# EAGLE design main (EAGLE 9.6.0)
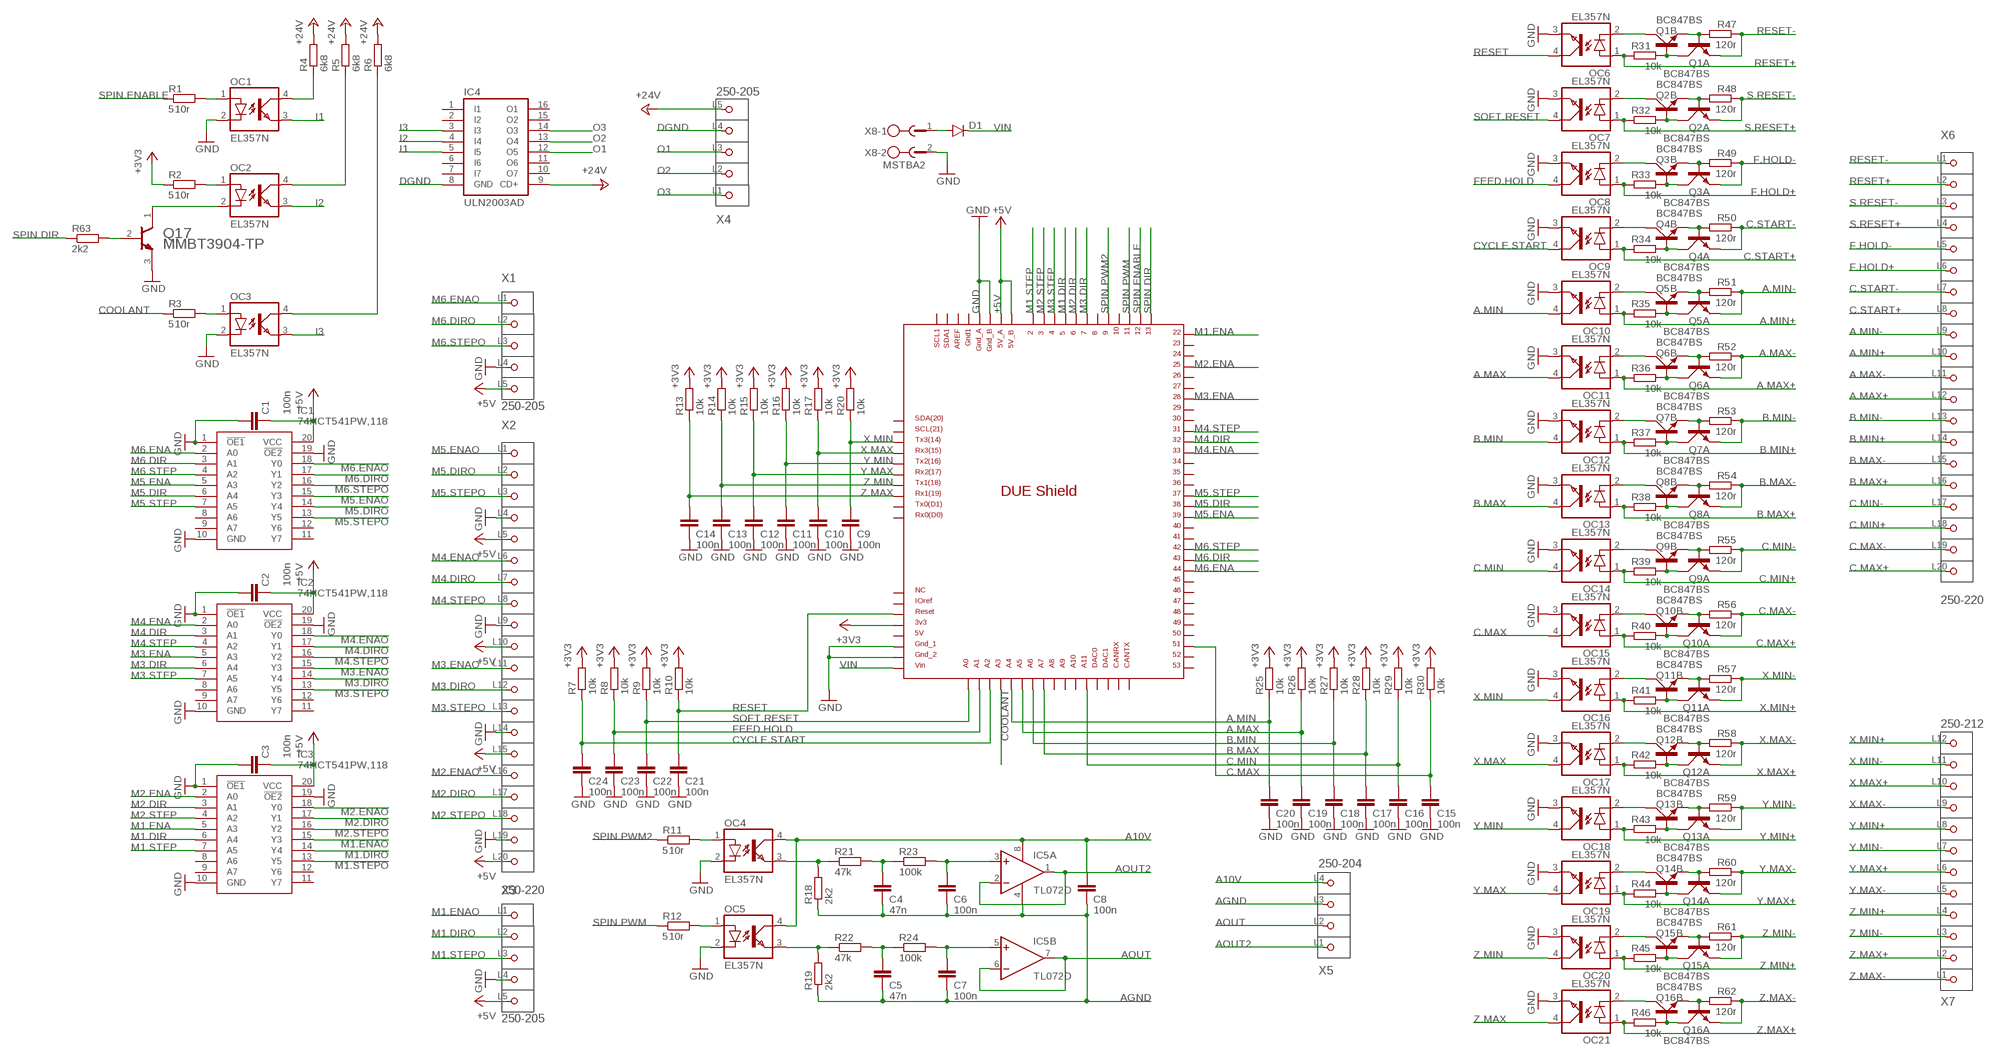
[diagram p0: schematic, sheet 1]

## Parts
C1  100n  CAP_0402  [0402]
C2  100n  CAP_0402  [0402]
C3  100n  CAP_0402  [0402]
C4  47n  CAP_0402  [0402]
C5  47n  CAP_0402  [0402]
C6  100n  CAP_0402  [0402]
C7  100n  CAP_0402  [0402]
C8  100n  CAP_0402  [0402]
C9  100n  CAP_0402  [0402]
C10  100n  CAP_0402  [0402]
C11  100n  CAP_0402  [0402]
C12  100n  CAP_0402  [0402]
C13  100n  CAP_0402  [0402]
C14  100n  CAP_0402  [0402]
C15  100n  CAP_0402  [0402]
C16  100n  CAP_0402  [0402]
C17  100n  CAP_0402  [0402]
C18  100n  CAP_0402  [0402]
C19  100n  CAP_0402  [0402]
C20  100n  CAP_0402  [0402]
C21  100n  CAP_0402  [0402]
C22  100n  CAP_0402  [0402]
C23  100n  CAP_0402  [0402]
C24  100n  CAP_0402  [0402]
D1  DIODE-DO214AC  [DO214AC]
IC1  74HCT541PW,118  [SOP65P640X110-20N]
IC2  74HCT541PW,118  [SOP65P640X110-20N]
IC3  74HCT541PW,118  [SOP65P640X110-20N]
IC4  ULN2003AD  [SO16]
IC5  TL072D  [SO08]
MCU1  DUE(NORMAL)  [DUE(NORMAL)]
OC1  EL357N  [SOP4]
OC2  EL357N  [SOP4]
OC3  EL357N  [SOP4]
OC4  EL357N  [SOP4]
OC5  EL357N  [SOP4]
OC6  EL357N  [SOP4]
OC7  EL357N  [SOP4]
OC8  EL357N  [SOP4]
OC9  EL357N  [SOP4]
OC10  EL357N  [SOP4]
OC11  EL357N  [SOP4]
OC12  EL357N  [SOP4]
OC13  EL357N  [SOP4]
OC14  EL357N  [SOP4]
OC15  EL357N  [SOP4]
OC16  EL357N  [SOP4]
OC17  EL357N  [SOP4]
OC18  EL357N  [SOP4]
OC19  EL357N  [SOP4]
OC20  EL357N  [SOP4]
OC21  EL357N  [SOP4]
Q1  BC847BS  [SOT363_PHILIPS]
Q2  BC847BS  [SOT363_PHILIPS]
Q3  BC847BS  [SOT363_PHILIPS]
Q4  BC847BS  [SOT363_PHILIPS]
Q5  BC847BS  [SOT363_PHILIPS]
Q6  BC847BS  [SOT363_PHILIPS]
Q7  BC847BS  [SOT363_PHILIPS]
Q8  BC847BS  [SOT363_PHILIPS]
Q9  BC847BS  [SOT363_PHILIPS]
Q10  BC847BS  [SOT363_PHILIPS]
Q11  BC847BS  [SOT363_PHILIPS]
Q12  BC847BS  [SOT363_PHILIPS]
Q13  BC847BS  [SOT363_PHILIPS]
Q14  BC847BS  [SOT363_PHILIPS]
Q15  BC847BS  [SOT363_PHILIPS]
Q16  BC847BS  [SOT363_PHILIPS]
Q17  MICRO_COMMERCIAL_MMBT3904-TPMICRO_COMMERCIAL_MMBT3904-TP_0_0  [MICRO_COMMERCIAL_MMBT3904-TP_0]
R1  510r  R-EU_R0402  [R0402]
R2  510r  R-EU_R0402  [R0402]
R3  510r  R-EU_R0402  [R0402]
R4  6k8  R-EU_R0603  [R0603]
R5  6k8  R-EU_R0603  [R0603]
R6  6k8  R-EU_R0603  [R0603]
R7  10k  R-EU_R0402  [R0402]
R8  10k  R-EU_R0402  [R0402]
R9  10k  R-EU_R0402  [R0402]
R10  10k  R-EU_R0402  [R0402]
R11  510r  R-EU_R0402  [R0402]
R12  510r  R-EU_R0402  [R0402]
R13  10k  R-EU_R0402  [R0402]
R14  10k  R-EU_R0402  [R0402]
R15  10k  R-EU_R0402  [R0402]
R16  10k  R-EU_R0402  [R0402]
R17  10k  R-EU_R0402  [R0402]
R18  2k2  R-EU_R0402  [R0402]
R19  2k2  R-EU_R0402  [R0402]
R20  10k  R-EU_R0402  [R0402]
R21  47k  R-EU_R0402  [R0402]
R22  47k  R-EU_R0402  [R0402]
R23  100k  R-EU_R0402  [R0402]
R24  100k  R-EU_R0402  [R0402]
R25  10k  R-EU_R0402  [R0402]
R26  10k  R-EU_R0402  [R0402]
R27  10k  R-EU_R0402  [R0402]
R28  10k  R-EU_R0402  [R0402]
R29  10k  R-EU_R0402  [R0402]
R30  10k  R-EU_R0402  [R0402]
R31  10k  R-EU_R0402  [R0402]
R32  10k  R-EU_R0402  [R0402]
R33  10k  R-EU_R0402  [R0402]
R34  10k  R-EU_R0402  [R0402]
R35  10k  R-EU_R0402  [R0402]
R36  10k  R-EU_R0402  [R0402]
R37  10k  R-EU_R0402  [R0402]
R38  10k  R-EU_R0402  [R0402]
R39  10k  R-EU_R0402  [R0402]
R40  10k  R-EU_R0402  [R0402]
R41  10k  R-EU_R0402  [R0402]
R42  10k  R-EU_R0402  [R0402]
R43  10k  R-EU_R0402  [R0402]
R44  10k  R-EU_R0402  [R0402]
R45  10k  R-EU_R0402  [R0402]
R46  10k  R-EU_R0402  [R0402]
R47  120r  R-EU_R0402  [R0402]
R48  120r  R-EU_R0402  [R0402]
R49  120r  R-EU_R0402  [R0402]
R50  120r  R-EU_R0402  [R0402]
R51  120r  R-EU_R0402  [R0402]
R52  120r  R-EU_R0402  [R0402]
R53  120r  R-EU_R0402  [R0402]
R54  120r  R-EU_R0402  [R0402]
R55  120r  R-EU_R0402  [R0402]
R56  120r  R-EU_R0402  [R0402]
R57  120r  R-EU_R0402  [R0402]
R58  120r  R-EU_R0402  [R0402]
R59  120r  R-EU_R0402  [R0402]
R60  120r  R-EU_R0402  [R0402]
R61  120r  R-EU_R0402  [R0402]
R62  120r  R-EU_R0402  [R0402]
R63  2k2  R-EU_R0402  [R0402]
X1  250-205  [P-250-205]
X2  250-220  [P-250-220]
X3  250-205  [P-250-205]
X4  250-205  [P-250-205]
X5  250-204  [P-250-204]
X6  250-220  [P-250-220]
X7  250-212  [P-250-212]
X8  MSTBA2  [MSTBA2]

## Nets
+3V3 [power1]: MCU1.3V3 R2.1 R7.2 R8.2 R9.2 R10.2 R13.2 R14.2 R15.2 R16.2 R17.2 R20.2 R25.2 R26.2 R27.2 R28.2 R29.2 R30.2
+5V [power1]: C1.2 C2.2 C3.2 IC1.20(VCC) IC2.20(VCC) IC3.20(VCC) MCU1.5V_A MCU1.5V_B X1.L5(P5) X2.L5(P5) X2.L10(P10) X2.L15(P15) X2.L20(P20) X3.L5(P5)
+24V [power1]: IC4.9(CD+) R4.2 R5.2 R6.2 X4.L5(P5)
A10V [signal1]: C8.1 IC5.8(P:V+) OC4.4(COL) OC5.4(COL) X5.L4(P4)
A.MAX [signal1]: C19.1 MCU1.A5 OC11.4(COL) R26.1
A.MAX+ [signal1]: OC11.1(A) R36.2 X6.L12(P12)
A.MAX- [signal1]: Q6.1(A:E) R52.1 X6.L11(P11)
A.MIN [signal1]: C20.1 MCU1.A4 OC10.4(COL) R25.1
A.MIN+ [signal1]: OC10.1(A) R35.2 X6.L10(P10)
A.MIN- [signal1]: Q5.1(A:E) R51.1 X6.L9(P9)
AGND [signal1]: C4.2 C5.2 C6.2 C7.2 C8.2 IC5.4(P:V-) R18.1 R19.1 X5.L3(P3)
AOUT [signal1]: IC5.6(B:-IN) IC5.7(B:OUT) X5.L2(P2)
AOUT2 [signal1]: IC5.1(A:OUT) IC5.2(A:-IN) X5.L1(P1)
B.MAX [signal1]: C17.1 MCU1.A7 OC13.4(COL) R28.1
B.MAX+ [signal1]: OC13.1(A) R38.2 X6.L16(P16)
B.MAX- [signal1]: Q8.1(A:E) R54.1 X6.L15(P15)
B.MIN [signal1]: C18.1 MCU1.A6 OC12.4(COL) R27.1
B.MIN+ [signal1]: OC12.1(A) R37.2 X6.L14(P14)
B.MIN- [signal1]: Q7.1(A:E) R53.1 X6.L13(P13)
C.MAX [signal1]: C15.1 MCU1.51 OC15.4(COL) R30.1
C.MAX+ [signal1]: OC15.1(A) R40.2 X6.L20(P20)
C.MAX- [signal1]: Q10.1(A:E) R56.1 X6.L19(P19)
C.MIN [signal1]: C16.1 MCU1.A11 OC14.4(COL) R29.1
C.MIN+ [signal1]: OC14.1(A) R39.2 X6.L18(P18)
C.MIN- [signal1]: Q9.1(A:E) R55.1 X6.L17(P17)
C.START+ [signal1]: OC9.1(A) R34.2 X6.L8(P8)
C.START- [signal1]: Q4.1(A:E) R50.1 X6.L7(P7)
COOLANT [signal1]: MCU1.A3 R3.1
CYCLE.START [signal1]: C24.1 MCU1.A2 OC9.4(COL) R7.1
DGND [power1]: IC4.8(GND) X4.L4(P4)
F.HOLD+ [signal1]: OC8.1(A) R33.2 X6.L6(P6)
F.HOLD- [signal1]: Q3.1(A:E) R49.1 X6.L5(P5)
FEED.HOLD [signal1]: C23.1 MCU1.A1 OC8.4(COL) R8.1
GND: C1.1 C2.1 C3.1 C9.2 C10.2 C11.2 C12.2 C13.2 C14.2 C15.2 C16.2 C17.2 C18.2 C19.2 C20.2 C21.2 C22.2 C23.2 C24.2 IC1.1(!OE1) IC1.10(GND) IC1.19(!OE2) IC2.1(!OE1) IC2.10(GND) IC2.19(!OE2) IC3.1(!OE1) IC3.10(GND) IC3.19(!OE2) MCU1.GND_1 MCU1.GND_2 MCU1.GND_A MCU1.GND_B OC1.2(C) OC3.2(C) OC4.2(C) OC5.2(C) OC6.3(EMIT) OC7.3(EMIT) OC8.3(EMIT) OC9.3(EMIT) OC10.3(EMIT) OC11.3(EMIT) OC12.3(EMIT) OC13.3(EMIT) OC14.3(EMIT) OC15.3(EMIT) OC16.3(EMIT) OC17.3(EMIT) OC18.3(EMIT) OC19.3(EMIT) OC20.3(EMIT) OC21.3(EMIT) Q17.3(E) X1.L4(P4) X2.L4(P4) X2.L9(P9) X2.L14(P14) X2.L19(P19) X3.L4(P4) X8.2
I1 [signal1]: IC4.5(I5) OC1.3(EMIT)
I2 [signal1]: IC4.4(I4) OC2.3(EMIT)
I3 [signal1]: IC4.3(I3) OC3.3(EMIT)
M1.DIR [signal1]: IC3.6(A4) MCU1.5
M1.DIRO [signal1]: IC3.14(Y4) X3.L2(P2)
M1.ENA [signal1]: IC3.5(A3) MCU1.22
M1.ENAO [signal1]: IC3.15(Y3) X3.L1(P1)
M1.STEP [signal1]: IC3.7(A5) MCU1.2
M1.STEPO [signal1]: IC3.13(Y5) X3.L3(P3)
M2.DIR [signal1]: IC3.3(A1) MCU1.6
M2.DIRO [signal1]: IC3.17(Y1) X2.L17(P17)
M2.ENA [signal1]: IC3.2(A0) MCU1.25
M2.ENAO [signal1]: IC3.18(Y0) X2.L16(P16)
M2.STEP [signal1]: IC3.4(A2) MCU1.3
M2.STEPO [signal1]: IC3.16(Y2) X2.L18(P18)
M3.DIR [signal1]: IC2.6(A4) MCU1.7
M3.DIRO [signal1]: IC2.14(Y4) X2.L12(P12)
M3.ENA [signal1]: IC2.5(A3) MCU1.28
M3.ENAO [signal1]: IC2.15(Y3) X2.L11(P11)
M3.STEP [signal1]: IC2.7(A5) MCU1.4
M3.STEPO [signal1]: IC2.13(Y5) X2.L13(P13)
M4.DIR [signal1]: IC2.3(A1) MCU1.32
M4.DIRO [signal1]: IC2.17(Y1) X2.L7(P7)
M4.ENA [signal1]: IC2.2(A0) MCU1.33
M4.ENAO [signal1]: IC2.18(Y0) X2.L6(P6)
M4.STEP [signal1]: IC2.4(A2) MCU1.31
M4.STEPO [signal1]: IC2.16(Y2) X2.L8(P8)
M5.DIR [signal1]: IC1.6(A4) MCU1.38
M5.DIRO [signal1]: IC1.14(Y4) X2.L2(P2)
M5.ENA [signal1]: IC1.5(A3) MCU1.39
M5.ENAO [signal1]: IC1.15(Y3) X2.L1(P1)
M5.STEP [signal1]: IC1.7(A5) MCU1.37
M5.STEPO [signal1]: IC1.13(Y5) X2.L3(P3)
M6.DIR [signal1]: IC1.3(A1) MCU1.43
M6.DIRO [signal1]: IC1.17(Y1) X1.L2(P2)
M6.ENA [signal1]: IC1.2(A0) MCU1.44
M6.ENAO [signal1]: IC1.18(Y0) X1.L1(P1)
M6.STEP [signal1]: IC1.4(A2) MCU1.42
M6.STEPO [signal1]: IC1.16(Y2) X1.L3(P3)
N$2 [signal1]: Q16.5(B:B) Q16.6(A:C) R46.1
N$3 [signal1]: Q16.2(A:B) Q16.4(B:E) R62.2
N$4 [signal1]: OC21.2(C) Q16.3(B:C)
N$5 [signal1]: Q15.5(B:B) Q15.6(A:C) R45.1
N$6 [signal1]: Q15.2(A:B) Q15.4(B:E) R61.2
N$7 [signal1]: OC20.2(C) Q15.3(B:C)
N$8 [signal1]: Q14.5(B:B) Q14.6(A:C) R44.1
N$9 [signal1]: Q14.2(A:B) Q14.4(B:E) R60.2
N$10 [signal1]: OC19.2(C) Q14.3(B:C)
N$11 [signal1]: Q13.5(B:B) Q13.6(A:C) R43.1
N$12 [signal1]: Q13.2(A:B) Q13.4(B:E) R59.2
N$13 [signal1]: OC18.2(C) Q13.3(B:C)
N$14 [signal1]: Q12.5(B:B) Q12.6(A:C) R42.1
N$15 [signal1]: Q12.2(A:B) Q12.4(B:E) R58.2
N$16 [signal1]: OC17.2(C) Q12.3(B:C)
N$17 [signal1]: Q11.5(B:B) Q11.6(A:C) R41.1
N$18 [signal1]: Q11.2(A:B) Q11.4(B:E) R57.2
N$19 [signal1]: OC15.2(C) Q10.3(B:C)
N$20 [signal1]: Q10.5(B:B) Q10.6(A:C) R40.1
N$21 [signal1]: Q10.2(A:B) Q10.4(B:E) R56.2
N$22 [signal1]: OC16.2(C) Q11.3(B:C)
N$23 [signal1]: Q4.5(B:B) Q4.6(A:C) R34.1
N$24 [signal1]: Q9.5(B:B) Q9.6(A:C) R39.1
N$25 [signal1]: Q9.2(A:B) Q9.4(B:E) R55.2
N$26 [signal1]: OC4.3(EMIT) R18.2 R21.1
N$27 [signal1]: C5.1 R22.2 R24.1
N$28 [signal1]: OC14.2(C) Q9.3(B:C)
N$29 [signal1]: Q8.5(B:B) Q8.6(A:C) R38.1
N$30 [signal1]: Q8.2(A:B) Q8.4(B:E) R54.2
N$31 [signal1]: C4.1 R21.2 R23.1
N$32 [signal1]: C6.1 IC5.3(A:+IN) R23.2
N$33 [signal1]: OC13.2(C) Q8.3(B:C)
N$34 [signal1]: Q7.5(B:B) Q7.6(A:C) R37.1
N$35 [signal1]: Q7.2(A:B) Q7.4(B:E) R53.2
N$36 [signal1]: C7.1 IC5.5(B:+IN) R24.2
N$37 [signal1]: OC4.1(A) R11.2
N$38 [signal1]: OC12.2(C) Q7.3(B:C)
N$39 [signal1]: Q6.5(B:B) Q6.6(A:C) R36.1
N$40 [signal1]: Q6.2(A:B) Q6.4(B:E) R52.2
N$41 [signal1]: OC5.3(EMIT) R19.2 R22.1
N$42 [signal1]: OC5.1(A) R12.2
N$43 [signal1]: OC11.2(C) Q6.3(B:C)
N$44 [signal1]: Q5.5(B:B) Q5.6(A:C) R35.1
N$45 [signal1]: Q5.2(A:B) Q5.4(B:E) R51.2
N$46 [signal1]: Q4.2(A:B) Q4.4(B:E) R50.2
N$47 [signal1]: OC9.2(C) Q4.3(B:C)
N$48 [signal1]: OC10.2(C) Q5.3(B:C)
N$49 [signal1]: Q3.5(B:B) Q3.6(A:C) R33.1
N$50 [signal1]: Q3.2(A:B) Q3.4(B:E) R49.2
N$51 [signal1]: OC8.2(C) Q3.3(B:C)
N$52 [signal1]: Q2.5(B:B) Q2.6(A:C) R32.1
N$53 [signal1]: Q2.2(A:B) Q2.4(B:E) R48.2
N$54 [signal1]: OC7.2(C) Q2.3(B:C)
N$55 [signal1]: Q1.5(B:B) Q1.6(A:C) R31.1
N$56 [signal1]: Q1.2(A:B) Q1.4(B:E) R47.2
N$57 [signal1]: OC6.2(C) Q1.3(B:C)
N$58 [signal1]: OC1.1(A) R1.2
N$59 [signal1]: OC2.1(A) R2.2
N$60 [signal1]: OC3.1(A) R3.2
N$61 [signal1]: OC1.4(COL) R4.1
N$62 [signal1]: OC2.4(COL) R5.1
N$63 [signal1]: OC3.4(COL) R6.1
N$64: OC2.2(C) Q17.1(C)
N$65: Q17.2(B) R63.2
N$66 [power1]: D1.A X8.1
O1 [power1]: IC4.12(O5) X4.L3(P3)
O2 [power1]: IC4.13(O4) X4.L2(P2)
O3 [power1]: IC4.14(O3) X4.L1(P1)
RESET [signal1]: C21.1 MCU1.RESET OC6.4(COL) R10.1
RESET+ [signal1]: OC6.1(A) R31.2 X6.L2(P2)
RESET- [signal1]: Q1.1(A:E) R47.1 X6.L1(P1)
S.RESET+ [signal1]: OC7.1(A) R32.2 X6.L4(P4)
S.RESET- [signal1]: Q2.1(A:E) R48.1 X6.L3(P3)
SOFT.RESET [signal1]: C22.1 MCU1.A0 OC7.4(COL) R9.1
SPIN.DIR [signal1]: MCU1.13 R63.1
SPIN.ENABLE [signal1]: MCU1.12 R1.1
SPIN.PWM [signal1]: MCU1.11 R12.1
SPIN.PWM2 [signal1]: MCU1.9 R11.1
VIN [power1]: D1.C MCU1.VIN
X.MAX [signal1]: C10.1 MCU1.RX3 OC17.4(COL) R17.1
X.MAX+ [signal1]: OC17.1(A) R42.2 X7.L10(P10)
X.MAX- [signal1]: Q12.1(A:E) R58.1 X7.L9(P9)
X.MIN [signal1]: C9.1 MCU1.TX3 OC16.4(COL) R20.1
X.MIN+ [signal1]: OC16.1(A) R41.2 X7.L12(P12)
X.MIN- [signal1]: Q11.1(A:E) R57.1 X7.L11(P11)
Y.MAX [signal1]: C12.1 MCU1.RX2 OC19.4(COL) R15.1
Y.MAX+ [signal1]: OC19.1(A) R44.2 X7.L6(P6)
Y.MAX- [signal1]: Q14.1(A:E) R60.1 X7.L5(P5)
Y.MIN [signal1]: C11.1 MCU1.TX2 OC18.4(COL) R16.1
Y.MIN+ [signal1]: OC18.1(A) R43.2 X7.L8(P8)
Y.MIN- [signal1]: Q13.1(A:E) R59.1 X7.L7(P7)
Z.MAX [signal1]: C14.1 MCU1.RX1 OC21.4(COL) R13.1
Z.MAX+ [signal1]: OC21.1(A) R46.2 X7.L2(P2)
Z.MAX- [signal1]: Q16.1(A:E) R62.1 X7.L1(P1)
Z.MIN [signal1]: C13.1 MCU1.TX1 OC20.4(COL) R14.1
Z.MIN+ [signal1]: OC20.1(A) R45.2 X7.L4(P4)
Z.MIN- [signal1]: Q15.1(A:E) R61.1 X7.L3(P3)
Unconnected: IC1.8(A6) IC1.9(A7) IC1.11(Y7) IC1.12(Y6) IC2.8(A6) IC2.9(A7) IC2.11(Y7) IC2.12(Y6) IC3.8(A6) IC3.9(A7) IC3.11(Y7) IC3.12(Y6) IC4.1(I1) IC4.2(I2) IC4.6(I6) IC4.7(I7) IC4.10(O7) IC4.11(O6) IC4.15(O2) IC4.16(O1) MCU1.5V MCU1.8 MCU1.10 MCU1.23 MCU1.24 MCU1.26 MCU1.27 MCU1.29 MCU1.30 MCU1.34 MCU1.35 MCU1.36 MCU1.40 MCU1.41 MCU1.45 MCU1.46 MCU1.47 MCU1.48 MCU1.49 MCU1.50 MCU1.52 MCU1.53 MCU1.A8 MCU1.A9 MCU1.A10 MCU1.AREF MCU1.CANRX MCU1.CANTX MCU1.DAC0 MCU1.DAC1 MCU1.GND1 MCU1.IOREF MCU1.NC MCU1.RX0 MCU1.SCL MCU1.SCL1 MCU1.SDA MCU1.SDA1 MCU1.TX0

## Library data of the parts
C1-C24 = Perfect_0402:CAP_0402: 0402 (1005 Metric)
D1 = mydiode:DIODE-: DIODE
IC1-IC3 = SamacSys_Parts:74HCT541PW,118: 74HC(T)541 - Octal buffer/line driver; 3-state@en-us Source: Datasheet; DESCRIPTION: 74HC(T)541 - Octal buffer/line driver; 3-state@en-us; HEIGHT: 1.1mm; MANUFACTURER_NAME: Nexperia; MANUFACTURER_PART_NUMBER: 74HCT541PW,118; MOUSER_PART_NUMBER: 771-74HCT541PW-T; MOUSER_PRICE-STOCK: https://www.mouser.com/Search/Refine.aspx?Keyword=771-74HCT541PW-T
IC4 = uln-udn:ULN2003A: DRIVER ARRAY
IC5 = linear:TL072: OP AMP
MCU1 = DUElib130425:DUE(NORMAL)
OC1-OC21 = el357n:EL357N
Q1-Q16 = transistor-small-signal:BC847BS: NPN general purpose double transistor Source: http://www.farnell.com/datasheets/2466.pdf
Q17 = Micro Commercial - MMBT3904-TP:MICRO_COMMERCIAL_MMBT3904-TP: TRANS NPN 40V 0.2A SOT23; CENTROID_NOT_SPECIFIED: No; COLLECTOR_EMITTER_BREAKDOWN_VOLTAGE: 40V; COLLECTOR_EMITTER_SATURATION_VOLTAGE: 0.2V; DATASHEET: http://www.mccsemi.com/up_pdf/MMBT3904(SOT-23)-F.pdf; DEVICE_CLASS_L1: Discrete Semiconductors; DEVICE_CLASS_L2: Transistors; DEVICE_CLASS_L3: BJTs; DIGIKEY_DESCRIPTION: TRANS NPN 40V 0.2A SOT23; DIGIKEY_PART_NUMBER: MMBT3904TPMSCT-ND; GAIN_BANDWIDTH_PRODUCT: 300MHz; HEIGHT: 1.12mm; HFE_MIN: 100; LEAD_FREE: yes; MAX_COLLECTOR_CURRENT: 200mA; MAX_JUNCTION_TEMP: +150°C; MF: Micro Commercial; MFG_PACKAGE_IDENT: SOT-23; MFG_PACKAGE_IDENT_DATE: 0; MFG_PACKAGE_IDENT_REV: 0; MOUSER_DESCRIPTION: Bipolar Transistors - BJT 40V; MOUSER_PART_NUMBER: 833-MMBT3904-TP; MPN: MMBT3904-TP; NUMBER_OF_ELEMENTS: 1; NUMBER_OF_NPN: 1; NUMBER_OF_PNP: 0; PACKAGE: SOT23-3; POWER_DISSIPATION: 350mW; PREFIX: Q; ROHS: yes; STANDOFF_HEIGHT: 0.013mm; TEMPERATURE_RANGE_HIGH: +150°C; TEMPERATURE_RANGE_LOW: -55°C; VERIFICATION_VERSION: 0.0.0.1
R1-R63 = rcl:R-EU_: RESISTOR, European symbol; SPICEPREFIX: R
X1 X3 X4 = con-wago_250:250-205: Serie 250, 1-Leiter-Klemmenleiste für Leiterplatten 1 Lötstift/Pol versetzt / Series 250, 1-conductor PCB terminal strip 1 solder pin/pole, staggered Polzahl / Pole No.: 5 Rastermaß / Pitch: 3.5 - 3.5 mm Bemessungsspannung / Rated Voltage: 320 V Nennstrom / Nominal Current: 8 A Leiterquerschnitt /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
X2 X6 = con-wago_250:250-220: Serie 250, 1-Leiter-Klemmenleiste für Leiterplatten 1 Lötstift/Pol versetzt / Series 250, 1-conductor PCB terminal strip 1 solder pin/pole, staggered Polzahl / Pole No.: 20 Rastermaß / Pitch: 3.5 - 3.5 mm Bemessungsspannung / Rated Voltage: 320 V Nennstrom / Nominal Current: 8 A Leiterquerschnitt /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
X5 = con-wago_250:250-204: Serie 250, 1-Leiter-Klemmenleiste für Leiterplatten 1 Lötstift/Pol versetzt / Series 250, 1-conductor PCB terminal strip 1 solder pin/pole, staggered Polzahl / Pole No.: 4 Rastermaß / Pitch: 3.5 - 3.5 mm Bemessungsspannung / Rated Voltage: 320 V Nennstrom / Nominal Current: 8 A Leiterquerschnitt /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
X7 = con-wago_250:250-212: Serie 250, 1-Leiter-Klemmenleiste für Leiterplatten 1 Lötstift/Pol versetzt / Series 250, 1-conductor PCB terminal strip 1 solder pin/pole, staggered Polzahl / Pole No.: 12 Rastermaß / Pitch: 3.5 - 3.5 mm Bemessungsspannung / Rated Voltage: 320 V Nennstrom / Nominal Current: 8 A Leiterquerschnitt /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
X8 = con-phoenix-508:MSTBA2: PHOENIX; MF: FARNELL; MPN: 1757242; OC_FARNELL: 3705171; OC_NEWARK: 71C4161

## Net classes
0 default: clearance 0.254 mm
1 power1: width 0.457 mm
2 signal1: width 0.305 mm

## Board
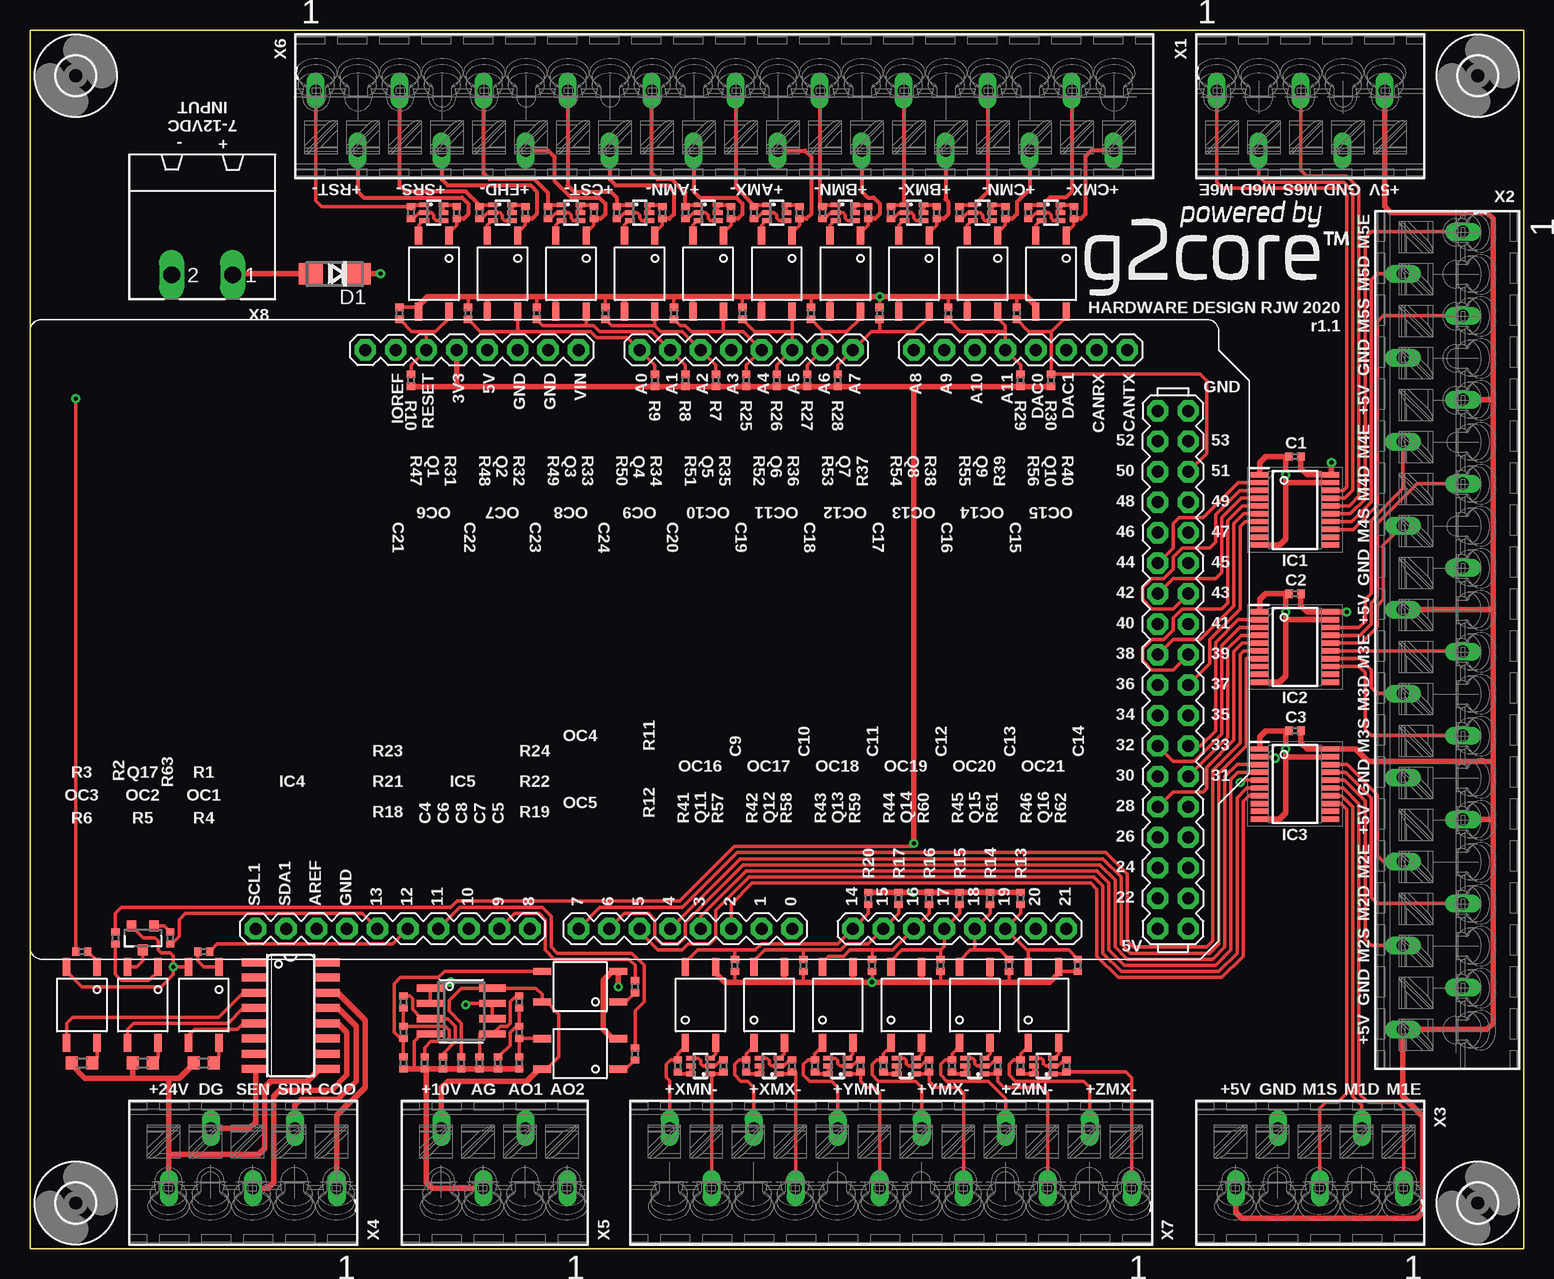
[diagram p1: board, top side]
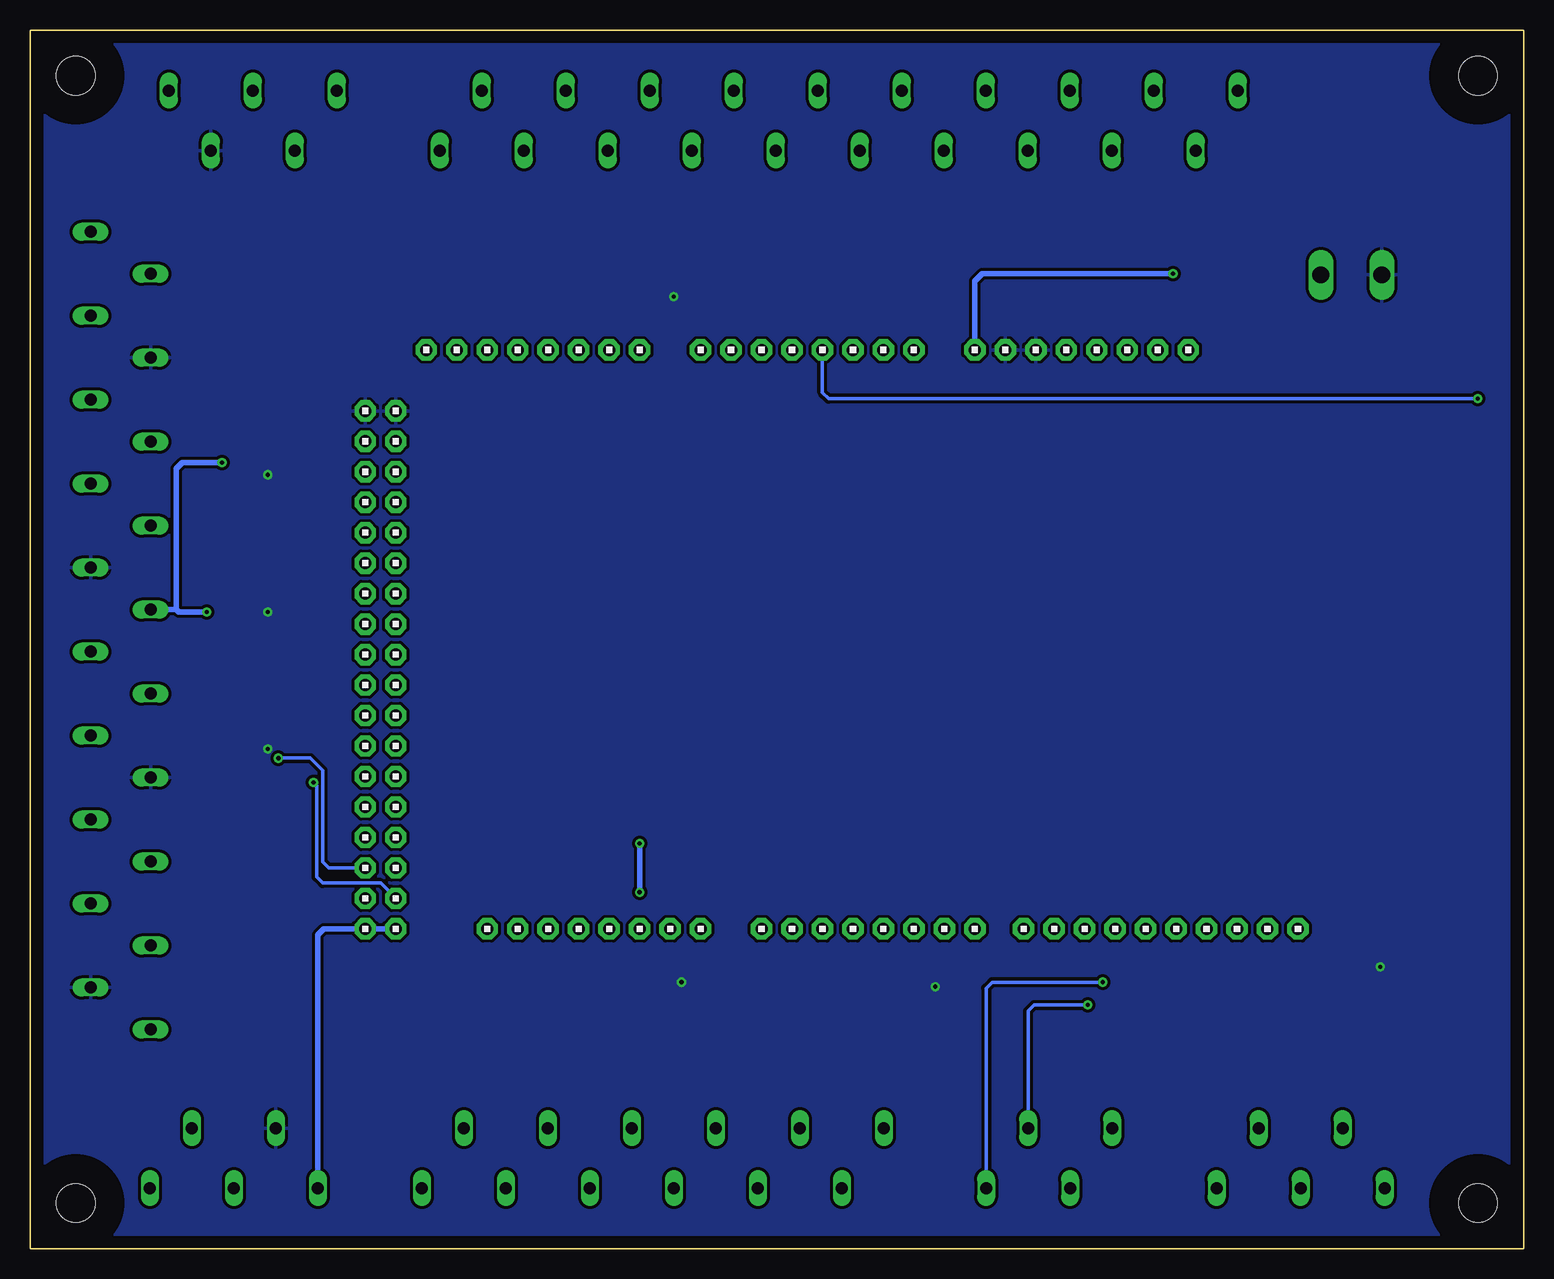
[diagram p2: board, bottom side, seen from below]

Size 124.46 x 101.6 mm. Coordinates in mm from the lower left corner, seen from the top.
Outline: 0,101.6 124.46,101.6 124.46,0 0,0 0,101.6
Copper layers (1*16): Top 0.035mm / dielectric 1.5mm / Bottom 0.035mm
Design rules "default *": minimum track width 6mil, minimum drill 0.35mm, track to track 6mil, track to pad 6mil, pad to pad 6mil, via to via 6mil, smd to smd 6mil, copper to edge 40mil, drill to drill 6mil, minimum pad ring 10mil, minimum via ring 8mil, stop-mask expansion 4mil, vias tented up to drill 20mil, thermal gap 10mil

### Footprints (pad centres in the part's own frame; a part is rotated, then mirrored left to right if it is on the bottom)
0402 = smd 0.6 x 0.7: 1 -0.5,0; 2 0.5,0
DO214AC = smd 2 x 1.8: A 2,0; C -2,0
SOP65P640X110-20N = smd 1.475 x 0.45: 1 -2.938,2.925; 2 -2.938,2.275; 3 -2.938,1.625; 4 -2.938,0.975; 5 -2.938,0.325; 6 -2.938,-0.325; 7 -2.938,-0.975; 8 -2.938,-1.625; 9 -2.938,-2.275; 10 -2.938,-2.925; 11 2.938,-2.925; 12 2.938,-2.275; 13 2.938,-1.625; 14 2.938,-0.975; 15 2.938,-0.325; 16 2.938,0.325; 17 2.938,0.975; 18 2.938,1.625; 19 2.938,2.275; 20 2.938,2.925
SO16 = smd 0.66 x 2.032: 1 -4.445,-3.073; 2 -3.175,-3.073; 3 -1.905,-3.073; 4 -0.635,-3.073; 5 0.635,-3.073; 6 1.905,-3.073; 7 3.175,-3.073; 8 4.445,-3.073; 9 4.445,3.073; 10 3.175,3.073; 11 1.905,3.073; 12 0.635,3.073; 13 -0.635,3.073; 14 -1.905,3.073; 15 -3.175,3.073; 16 -4.445,3.073
SO08 = smd 0.6 x 2.2: 1 -1.905,-2.6; 2 -0.635,-2.6; 3 0.635,-2.6; 4 1.905,-2.6; 5 1.905,2.6; 6 0.635,2.6; 7 -0.635,2.6; 8 -1.905,2.6
DUE(NORMAL) = drill 1 pad 1.778 octagon: 2 43.18,50.8; 3 45.72,50.8; 3V3 66.04,2.54; 4 48.26,50.8; 5 50.8,50.8; 5V 63.5,2.54; 5V_A 7.62,50.8; 5V_B 5.08,50.8; 6 53.34,50.8; 7 55.88,50.8; 8 59.944,50.8; 9 62.484,50.8; 10 65.024,50.8; 11 67.564,50.8; 12 70.104,50.8; 13 72.644,50.8; 22 7.62,48.26; 23 5.08,48.26; 24 7.62,45.72; 25 5.08,45.72; 26 7.62,43.18; 27 5.08,43.18; 28 7.62,40.64; 29 5.08,40.64; 30 7.62,38.1; 31 5.08,38.1; 32 7.62,35.56; 33 5.08,35.56; 34 7.62,33.02; 35 5.08,33.02; 36 7.62,30.48; 37 5.08,30.48; 38 7.62,27.94; 39 5.08,27.94; 40 7.62,25.4; 41 5.08,25.4; 42 7.62,22.86; 43 5.08,22.86; 44 7.62,20.32; 45 5.08,20.32; 46 7.62,17.78; 47 5.08,17.78; 48 7.62,15.24; 49 5.08,15.24; 50 7.62,12.7; 51 5.08,12.7; 52 7.62,10.16; 53 5.08,10.16; A0 50.8,2.54; A1 48.26,2.54; A2 45.72,2.54; A3 43.18,2.54; A4 40.64,2.54; A5 38.1,2.54; A6 35.56,2.54; A7 33.02,2.54; A8 27.94,2.54; A9 25.4,2.54; A10 22.86,2.54; A11 20.32,2.54; AREF 77.724,50.8; CANRX 12.7,2.54; CANTX 10.16,2.54; DAC0 17.78,2.54; DAC1 15.24,2.54; GND1 75.184,50.8; GND_1 60.96,2.54; GND_2 58.42,2.54; GND_A 7.62,7.62; GND_B 5.08,7.62; IOREF 71.12,2.54; NC 73.66,2.54; RESET 68.58,2.54; RX0 38.1,50.8; RX1 20.32,50.8; RX2 25.4,50.8; RX3 30.48,50.8; SCL 15.24,50.8; SCL1 82.804,50.8; SDA 17.78,50.8; SDA1 80.264,50.8; TX0 40.64,50.8; TX1 22.86,50.8; TX2 27.94,50.8; TX3 33.02,50.8; VIN 55.88,2.54
SOP4 = smd 0.61 x 1.499: 1 -1.27,-3.175; 2 1.27,-3.175; 3 1.27,3.175; 4 -1.27,3.175
SOT363_PHILIPS = smd 0.4 x 0.8: 1 -0.65,-0.8; 2 0,-0.8; 3 0.65,-0.8; 4 0.65,0.8; 5 0,0.8; 6 -0.65,0.8
MICRO_COMMERCIAL_MMBT3904-TP_0 = smd 0.8 x 0.9: 1 0,1; 2 -0.95,-1; 3 0.95,-1
R0402 = smd 0.6 x 0.7: 1 -0.5,0; 2 0.5,0
R0603 = smd 1 x 1.1: 1 -0.85,0; 2 0.85,0
3,2 = hole 3.2: 0,0
P-250-205 = drill 1 long: L1 1.3,7.8; L2 -3.7,4.3; L3 1.3,0.8; L4 -3.7,-2.7; L5 1.3,-6.2
P-250-220 = drill 1 long: L1 1.3,33.983; L2 -3.7,30.483; L3 1.3,26.983; L4 -3.7,23.483; L5 1.3,19.983; L6 -3.7,16.483; L7 1.3,12.982; L8 -3.7,9.482; L9 1.3,5.982; L10 -3.7,2.482; L11 1.3,-1.018; L12 -3.7,-4.518; L13 1.3,-8.018; L14 -3.7,-11.518; L15 1.3,-15.018; L16 -3.7,-18.517; L17 1.3,-22.017; L18 -3.7,-25.517; L19 1.3,-29.017; L20 -3.7,-32.517
P-250-204 = drill 1 long: L1 1.3,6.05; L2 -3.7,2.55; L3 1.3,-0.95; L4 -3.7,-4.45
P-250-212 = drill 1 long: L1 1.3,20.05; L2 -3.7,16.55; L3 1.3,13.05; L4 -3.7,9.55; L5 1.3,6.05; L6 -3.7,2.55; L7 1.3,-0.95; L8 -3.7,-4.45; L9 1.3,-7.95; L10 -3.7,-11.45; L11 1.3,-14.95; L12 -3.7,-18.45
MSTBA2 = drill 1.397 long: 1 -2.54,5.08; 2 2.54,5.08

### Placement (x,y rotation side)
C1  105.41,66.04 0 top
C2  105.41,54.61 0 top
C3  105.41,43.18 0 top
C4  32.89,15.49 270 top
C5  38.99,15.49 270 top
C6  34.42,15.49 270 top
C7  37.47,15.49 270 top
C8  35.94,15.49 270 top
C9  58.74,23.62 270 top
C10  64.45,23.62 270 top
C11  70.17,23.62 270 top
C12  75.88,23.62 270 top
C13  81.6,23.62 270 top
C14  87.31,23.62 270 top
C15  82.23,77.98 90 top
C16  76.52,77.98 90 top
C17  70.8,77.98 90 top
C18  65.09,77.98 90 top
C19  59.37,77.98 90 top
C20  53.66,77.98 90 top
C21  30.8,77.98 90 top
C22  36.51,77.98 90 top
C23  42.23,77.98 90 top
C24  47.94,77.98 90 top
D1  25.4,81.28 180 top
IC1  105.41,61.59 0 top
IC2  105.41,50.16 0 top
IC3  105.41,38.73 0 top
IC4  21.72,19.43 270 top
IC5  35.94,19.81 270 top
MCU1  101.6,77.47 180 top
OC1  14.48,20.32 180 top
OC2  9.4,20.32 180 top
OC3  4.32,20.32 180 top
OC4  45.85,21.84 90 top
OC5  45.85,16.26 90 top
OC6  33.66,81.28 180 top
OC7  39.37,81.28 180 top
OC8  45.09,81.28 180 top
OC9  50.8,81.28 180 top
OC10  56.52,81.28 180 top
OC11  62.23,81.28 180 top
OC12  67.94,81.28 180 top
OC13  73.66,81.28 180 top
OC14  79.38,81.28 180 top
OC15  85.09,81.28 180 top
OC16  55.88,20.32 0 top
OC17  61.59,20.32 0 top
OC18  67.31,20.32 0 top
OC19  73.03,20.32 0 top
OC20  78.74,20.32 0 top
OC21  84.45,20.32 0 top
Q1  33.66,86.36 270 top
Q2  39.37,86.36 270 top
Q3  45.09,86.36 270 top
Q4  50.8,86.36 270 top
Q5  56.52,86.36 270 top
Q6  62.23,86.36 270 top
Q7  67.94,86.36 270 top
Q8  73.66,86.36 270 top
Q9  79.38,86.36 270 top
Q10  85.09,86.36 270 top
Q11  55.88,15.24 90 top
Q12  61.59,15.24 90 top
Q13  67.31,15.24 90 top
Q14  73.03,15.24 90 top
Q15  78.74,15.24 90 top
Q16  84.45,15.24 90 top
Q17  9.4,25.91 180 top
R1  14.48,24.77 180 top
R2  7.11,25.91 270 top
R3  4.32,24.77 0 top
R4  14.48,15.49 180 top
R5  9.4,15.49 180 top
R6  4.32,15.49 180 top
R7  57.15,72.39 270 top
R8  54.61,72.39 270 top
R9  52.07,72.39 270 top
R10  31.75,72.39 270 top
R11  50.42,21.84 270 top
R12  50.42,16.26 270 top
R13  82.55,29.21 90 top
R14  80.01,29.21 90 top
R15  77.47,29.21 90 top
R16  74.93,29.21 90 top
R17  72.39,29.21 90 top
R18  31.11,15.49 90 top
R19  40.77,15.49 90 top
R20  69.85,29.21 90 top
R21  31.11,18.03 90 top
R22  40.77,18.03 90 top
R23  31.11,20.57 90 top
R24  40.77,20.57 90 top
R25  59.69,72.39 270 top
R26  62.23,72.39 270 top
R27  64.77,72.39 270 top
R28  67.31,72.39 270 top
R29  82.55,72.39 270 top
R30  85.09,72.39 270 top
R31  35.56,86.36 270 top
R32  41.27,86.36 270 top
R33  46.99,86.36 270 top
R34  52.7,86.36 270 top
R35  58.42,86.36 270 top
R36  64.14,86.36 270 top
R37  69.85,86.36 270 top
R38  75.56,86.36 270 top
R39  81.28,86.36 270 top
R40  87,86.36 270 top
R41  53.98,15.24 90 top
R42  59.69,15.24 90 top
R43  65.41,15.24 90 top
R44  71.12,15.24 90 top
R45  76.83,15.24 90 top
R46  82.55,15.24 90 top
R47  31.75,86.36 270 top
R48  37.47,86.36 270 top
R49  43.18,86.36 270 top
R50  48.9,86.36 270 top
R51  54.61,86.36 270 top
R52  60.33,86.36 270 top
R53  66.04,86.36 270 top
R54  71.75,86.36 270 top
R55  77.47,86.36 270 top
R56  83.19,86.36 270 top
R57  57.78,15.24 90 top
R58  63.5,15.24 90 top
R59  69.22,15.24 90 top
R60  74.93,15.24 90 top
R61  80.64,15.24 90 top
R62  86.36,15.24 90 top
R63  11.68,25.91 90 top
U$1  [3,2]  3.81,97.79 0 top
U$2  [3,2]  120.65,97.79 0 top
U$3  [3,2]  3.81,3.81 0 top
U$4  [3,2]  120.65,3.81 0 top
X1  106.68,95.25 90 top
X2  118.11,50.8 0 top
X3  106.68,6.35 270 top
X4  17.78,6.35 270 top
X5  38.73,6.35 270 top
X6  57.78,95.25 90 top
X7  71.75,6.35 270 top
X8  14.35,86.27 180 top

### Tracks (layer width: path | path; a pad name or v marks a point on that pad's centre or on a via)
+3V3  (via drill 0.35)
  Top 0.305: R2.1 7.11,27.94 7.62,28.45 33.53,28.45 35.05,28.45 35.59,28.98 54.13,28.98 58.7,33.55 73.43,33.55 v73.66,33.78
  Top 0.457: v73.66,33.78 73.66,71.89 R30.2 R29.2 R28.2 R27.2 R26.2 R25.2 R7.2 R8.2 R9.2 35.56,71.89 | R20.2 R17.2 v73.66,29.72 R16.2 R15.2 R14.2 R13.2 | R10.2 35.56,71.89 | 35.56,71.89 MCU1.3V3
  Bottom 0.457: v73.66,33.78 v73.66,29.72
+5V  (via drill 0.35)
  Top 0.457: v109.73,53.09 IC2.20 | IC2.20 | X3.L5 100.48,3.05 100.99,2.54 115.57,2.54 116.08,3.05 116.08,11.03 114.41,12.7 X2.L20 121.41,18.28 121.92,18.79 121.92,35.78 | 121.92,70.78 121.92,85.88 121.41,86.39 113.39,86.39 112.88,86.9 X1.L5 | 121.92,35.78 121.92,40.61 | 121.92,40.61 121.92,53.28 | 121.92,53.28 121.92,70.78 | X2.L5 121.92,70.78 | X2.L15 121.92,35.78 | 121.92,40.61 111.54,40.61 110.49,41.66 IC3.20 106.42,41.66 105.91,42.17 C3.2 | X2.L10 121.92,53.28 | C1.2 105.91,65.03 106.42,64.52 IC1.20 108.46,64.52 v108.46,65.53 | C2.2 105.91,53.59 106.42,53.09 IC2.20
  Bottom 0.457: X2.L10 112.27,53.28 | v108.46,65.53 111.76,65.53 112.27,65.02 112.27,53.28 | v109.73,53.09 112.07,53.09 112.27,53.28 | MCU1.5V_A MCU1.5V_B 99.97,26.67 100.48,26.16 X3.L5
+24V
  Top 0.457: R6.2 3.47,15.33 4.57,14.22 8.55,14.22 | R4.2 13.63,15.41 12.45,14.22 11.58,14.22 | 8.55,14.22 11.58,14.22 | R5.2 8.55,14.22 | X4.L5 11.58,7.87 | 11.58,7.87 11.58,14.22 | IC4.9 24.13,14.99 23.11,13.97 20.07,13.97 19.56,13.46 19.56,8.38 19.05,7.87 11.58,7.87
A10V
  Top 0.305: C8.1 35.94,18.8 34.92,19.81 34.92,20.7 35.94,21.72 IC5.8 42.16,21.72 42.67,21.21 OC4.4 43.05,20.57 44.07,19.56 44.07,16 43.05,14.99 OC5.4
  Top 0.457: X5.L4 34.28,13.46 34.79,13.97 41.4,13.97 42.42,14.99 OC5.4
A.MAX
  Top 0.305: R26.1 62.23,73.66 MCU1.A5 63.5,76.45 | OC11.4 63.5,76.45 | C19.1 60.4,76.45 63.5,76.45
A.MAX+
  Top 0.305: R36.2 64.14,85.34 63.5,84.71 OC11.1
  Top 0.318: X6.L12 64.58,91.55 65.09,91.04 65.09,86.24 64.71,85.86 R36.2
A.MAX-
  Top 0.305: R52.1 60.33,87.01 Q6.1
  Top 0.318: X6.L11 58.8,88.52 60.33,87 R52.1
A.MIN
  Top 0.305: R25.1 59.69,73.66 MCU1.A4 59.44,76.45 57.78,76.45 | C20.1 54.17,76.96 54.61,76.96 55.12,76.45 57.66,76.45 57.78,76.45 | OC10.4 57.78,76.45
A.MIN+
  Top 0.305: R35.2 58.42,85.34 57.78,84.71 OC10.1
  Top 0.318: X6.L10 55.3,88.14 55.81,87.63 58.86,87.63 59.37,87.12 59.37,86.24 58.99,85.86 R35.2
A.MIN-
  Top 0.305: R51.1 54.61,87.01 Q5.1
  Top 0.318: R51.1 54.61,88.01 53.47,89.15 52.31,89.15 51.8,89.66 X6.L9
AGND
  Top 0.305: IC5.4 32.64,17.91 32,17.27 32,14.99
  Top 0.457: C6.2 33.02,14.99 33.02,5.56 33.53,5.05 X5.L3 | C6.2 C4.2 32,14.99 R18.1 | C6.2 C8.2 C7.2 C5.2 R19.1
AOUT  (via drill 0.35)
  Top 0.305: v36.32,20.32 36.45,20.45 IC5.7 IC5.6
  Bottom 0.305: X5.L2 41.28,19.81 40.78,20.32 v36.32,20.32
AOUT2  (via drill 0.35)
  Top 0.305: v35.05,22.23 34.54,21.72 IC5.1 IC5.2
  Bottom 0.305: v35.05,22.23 44.28,22.23 44.78,21.72 X5.L1
B.MAX
  Top 0.305: R28.1 67.31,73.66 MCU1.A7 70.1,76.45 70.61,76.45 70.8,76.45 | OC13.4 74.93,77.72 73.66,76.45 70.8,76.45 | C17.1 70.8,76.45
B.MAX+
  Top 0.305: R38.2 75.56,85.34 74.93,84.71 OC13.1
  Top 0.318: X6.L16 76.3,87.49 76.52,87.27 76.52,86.24 76.14,85.86 R38.2
B.MAX-
  Top 0.305: R54.1 71.75,87.01 Q8.1
  Top 0.318: X6.L15 72.8,87.01 Q8.1
B.MIN
  Top 0.305: R27.1 64.77,73.66 MCU1.A6 66.04,76.53 | C18.1 65.95,76.62 66.04,76.53 | 66.04,76.53 66.11,76.45 68.07,76.45 69.22,77.6 OC12.4
B.MIN+
  Top 0.305: R37.2 69.85,85.34 69.22,84.71 OC12.1
  Top 0.318: X6.L14 69.3,88.14 69.81,87.63 70.29,87.63 70.8,87.12 70.8,86.24 70.42,85.86 R37.2
B.MIN-
  Top 0.305: R53.1 66.04,87.01 Q7.1
  Top 0.318: X6.L13 65.8,86.86 R53.1
C.MAX
  Top 0.305: MCU1.51 98.04,66.29 98.04,72.39 97.54,72.9 R30.1 | R30.1 | OC15.4 86.36,77.72 85.1,76.46 | 85.1,76.46 R30.1 | C15.1 83.25,76.46 85.1,76.46
C.MAX+
  Top 0.305: R40.2 87,85.34 86.36,84.71 OC15.1
  Top 0.318: X6.L20 88.46,91.55 87.95,91.04 87.95,86.24 87.57,85.86 R40.2
C.MAX-
  Top 0.305: R56.1 83.19,87.01 Q10.1
  Top 0.318: X6.L19 86.8,88.14 86.29,87.63 84.99,87.63 84.37,87.01 Q10.1
C.MIN
  Top 0.305: R29.1 82.55,73.66 MCU1.A11 81.28,76.45 | OC14.4 80.64,77.6 81.28,76.96 81.28,76.45 | C16.1 77.54,76.45 81.28,76.45
C.MIN+
  Top 0.305: R39.2 81.28,85.34 80.64,84.71 OC14.1
  Top 0.318: X6.L18 83.3,88.33 82.23,87.26 82.23,86.24 81.85,85.86 R39.2
C.MIN-
  Top 0.305: R55.1 77.47,87.01 Q9.1
  Top 0.318: X6.L17 79.8,88.14 78.67,87.01 Q9.1
C.START+
  Top 0.305: R34.2 52.7,85.34 52.07,84.71 OC9.1
  Top 0.318: X6.L8 48.3,89.15 48.81,88.65 53.15,88.65 53.66,88.14 53.66,86.24 53.28,85.86 R34.2
C.START-
  Top 0.305: R50.1 48.9,87.01 Q4.1
  Top 0.318: X6.L7 44.8,88.65 45.31,88.14 48.39,88.14 48.9,87.63 R50.1
COOLANT  (via drill 0.35)
  Top 0.305: v3.81,70.87 R3.1
  Bottom 0.305: v3.81,70.87 57.91,70.87 58.42,71.37 MCU1.A3
CYCLE.START
  Top 0.305: R7.1 57.15,73.66 MCU1.A2 54.36,76.45 52.58,76.45 52.07,76.96 | C24.1 48.46,76.96 52.07,76.96 | OC9.4 52.07,76.96
DGND
  Top 0.457: X4.L4 18.29,10.05 18.8,10.56 18.8,14.99 IC4.8
F.HOLD+
  Top 0.305: R33.2 46.99,85.34 46.35,84.71 OC8.1
  Top 0.318: X6.L6 43.18,91.55 43.69,91.04 43.69,89.03 45.09,87.63 47.43,87.63 47.94,87.12 47.94,86.24 47.56,85.86 R33.2
F.HOLD-
  Top 0.305: R49.1 43.18,87.01 Q3.1
  Top 0.318: R49.1 43.18,88.01 42.04,89.15 38.31,89.15 37.8,89.66 X6.L5
FEED.HOLD
  Top 0.305: R8.1 54.61,73.66 MCU1.A1 51.82,76.45 47.5,76.45 46.99,76.96 46.35,76.96 | C23.1 42.74,76.96 46.35,76.96 | OC8.4 46.35,76.96
GND  (via drill 0.35)
  Top 0.305: v11.94,23.5 11.94,24.4 11.68,24.65 10.92,24.65 10.67,24.91 10.67,25.65 10.41,25.91 9.45,25.91 Q17.3 | OC3.2 3.05,23.11 4.32,21.84 10.92,21.84 11.94,22.86 v11.94,23.5 | v11.94,23.5 OC1.2 | C9.2 58.74,22.23 58.8,22.23 | C10.2 64.45,22.23 64.52,22.23 | C11.2 v70.17,22.23 | C12.2 75.88,22.29 75.82,22.23 | C13.2 81.6,22.29 81.53,22.23 | C14.2 85.72,23.12 OC21.3 | C15.2 82.23,79.38 82.3,79.38 | C16.2 76.52,79.38 76.45,79.38 | C17.2 v70.8,79.38 | C18.2 65.09,79.38 65.02,79.38 | C19.2 59.37,79.38 59.44,79.38 | C20.2 53.66,79.38 53.59,79.38 | C24.2 47.94,79.38 48.01,79.38 | C23.2 42.23,79.38 42.16,79.38 | C22.2 36.51,79.38 36.58,79.38 | C21.2 32.38,78.48 OC6.3
  Top 0.457: OC16.3 57.15,22.99 57.91,22.23 58.8,22.23 62.87,22.23 | 80.01,22.23 81.53,22.23 84.96,22.23 85.72,22.99 OC21.3 | 62.87,22.23 64.52,22.23 68.58,22.23 | 68.58,22.23 v70.17,22.23 74.3,22.23 | 74.3,22.23 75.82,22.23 80.01,22.23 | OC17.3 62.87,22.23 | OC18.3 68.58,22.23 | OC19.3 74.3,22.23 | OC20.3 80.01,22.23 | OC15.3 83.82,78.61 83.06,79.38 82.3,79.38 78.11,79.38 | 78.11,79.38 76.45,79.38 72.39,79.38 | 72.39,79.38 v70.8,79.38 66.67,79.38 | OC10.3 55.24,79.38 | 55.24,79.38 59.44,79.38 60.96,79.38 | 60.96,79.38 65.02,79.38 66.67,79.38 | OC11.3 60.96,79.38 | OC12.3 66.67,79.38 | OC14.3 78.11,79.38 | OC13.3 72.39,79.38 | IC3.10 104.14,35.81 104.65,36.32 104.65,41.01 | IC3.19 104.65,41.01 | OC5.2 48.51,17.53 47.75,18.29 47.75,22.35 48.51,23.11 OC4.2 v49.02,21.84 | OC9.3 49.53,79.38 | 49.53,79.38 53.59,79.38 55.24,79.38 | OC8.3 43.81,79.38 | 43.81,79.38 48.01,79.38 49.53,79.38 | OC7.3 38.1,79.38 | 38.1,79.38 42.16,79.38 43.81,79.38 | OC6.3 32.38,78.61 33.15,79.38 36.58,79.38 38.1,79.38 | IC3.1 102.47,42.67 102.98,43.18 C3.1 104.65,43.18 v104.65,41.66 104.65,41.01 | IC1.10 104.14,58.67 104.65,59.18 v104.65,64.52 | IC1.19 104.65,63.87 v104.65,64.52 | IC1.1 102.47,65.53 102.98,66.04 C1.1 104.65,66.04 v104.65,64.52 | IC2.10 104.14,47.24 104.65,47.75 v104.65,53.09 | IC2.1 102.47,54.1 102.98,54.61 C2.1 104.65,54.61 v104.65,53.09 | IC2.19 104.65,52.44 v104.65,53.09
  pour Bottom: 0.64,100.97 123.83,100.97 123.83,0.64 0.64,0.64
I1
  Top 0.305: IC4.5 17.78,18.8 17.27,18.29 13.72,18.29 13.21,17.78 OC1.3
I2
  Top 0.305: IC4.4 17.78,20.07 16.51,18.8 8.64,18.8 8.13,18.29 OC2.3
I3
  Top 0.305: IC4.3 17.78,21.34 15.75,19.3 3.56,19.3 3.05,18.8 OC3.3
M1.DIR
  Top 0.305: MCU1.5 50.8,26.42 52.32,24.89 54.36,24.89 54.86,25.4 56.64,25.4 57.15,25.91 57.15,28.19 59.94,30.99 88.65,30.99 89.41,30.23 89.41,24.64 90.93,23.11 99.06,23.11 100.58,24.64 100.58,37.59 101.4,38.41 IC3.6
M1.DIRO
  Top 0.305: IC3.14 109.31,37.76 110.24,36.83 110.24,12.7 110.98,11.96 X3.L2
M1.ENA  (via drill 0.35)
  Top 0.305: IC3.5 101.04,39.06 v100.84,38.86
  Bottom 0.305: MCU1.22 95.25,30.48 100.08,30.48 100.58,30.99 100.58,38.61 v100.84,38.86
M1.ENAO
  Top 0.305: IC3.15 109.42,38.41 110.74,37.08 110.74,12.97 111.5,12.21 113.97,12.21 114.48,11.7 X3.L1
M1.STEP
  Top 0.305: MCU1.2 58.42,28.7 60.2,30.48 88.39,30.48 88.9,29.97 88.9,24.38 90.68,22.61 99.31,22.61 101.09,24.38 101.09,37.27 101.6,37.78 102.45,37.78 IC3.7
M1.STEPO
  Top 0.305: IC3.13 109.22,37.11 109.73,36.6 109.73,12.95 108.97,12.19 107.99,12.19 107.48,11.68 X3.L3
M2.DIR
  Top 0.305: MCU1.6 49.53,27.94 51.56,27.94 52.07,27.43 52.07,25.97 52.64,25.4 54.04,25.4 54.61,25.97 54.61,27.18 59.44,32 89.15,32 90.42,30.73 90.42,25.15 91.44,24.13 98.55,24.13 99.57,25.15 99.57,39.37 100.58,40.39 102.45,40.39 IC3.3
M2.DIRO
  Top 0.305: IC3.17 109.64,39.71 111.76,37.59 111.76,29.29 112.27,28.78 X2.L17
M2.ENA  (via drill 0.35)
  Top 0.305: IC3.2 103.64,41.01 v103.76,40.89
  Bottom 0.305: MCU1.25 99.57,31.75 100.08,32.26 100.08,39.88 101.09,40.89 v103.76,40.89
M2.ENAO
  Top 0.305: IC3.18 109.75,40.36 112.27,37.85 112.27,32.79 112.78,32.28 X2.L16
M2.STEP
  Top 0.305: MCU1.3 55.88,27.69 59.69,31.5 88.9,31.5 89.92,30.48 89.92,24.89 91.19,23.62 98.81,23.62 100.08,24.89 100.08,39.12 100.66,39.7 IC3.4
M2.STEPO
  Top 0.305: IC3.16 109.53,39.06 111.25,37.34 111.25,25.79 111.76,25.28 X2.L18
M3.DIR
  Top 0.305: IC2.6 101.15,49.84 100.84,49.53 100.84,42.16 98.55,39.88 98.55,25.65 98.04,25.15 91.95,25.15 91.44,25.65 91.44,31.24 89.66,33.02 58.93,33.02 54.36,28.45 47.5,28.45 MCU1.7
M3.DIRO
  Top 0.305: X2.L12 112.27,46.28 111.76,46.79 111.76,48.26 110.83,49.19 IC2.14
M3.ENA
  Top 0.305: MCU1.28 95.25,38.1 97.79,38.1 98.04,38.35 98.04,40.13 100.33,42.42 100.33,49.78 101.04,50.49 IC2.5
M3.ENAO
  Top 0.305: IC2.15 119.41,49.84 X2.L11
M3.STEP
  Top 0.305: MCU1.4 59.18,32.51 89.41,32.51 90.93,30.99 90.93,25.4 91.69,24.64 98.3,24.64 99.06,25.4 99.06,39.62 101.35,41.91 101.35,49.19 IC2.7
M3.STEPO
  Top 0.305: X2.L13 111.76,42.78 111.25,43.29 111.25,48.03 110.74,48.54 IC2.13
M4.DIR
  Top 0.305: MCU1.32 95.25,40.64 97.03,40.64 99.31,42.93 99.31,50.29 100.81,51.79 IC2.3
M4.DIRO
  Top 0.305: IC2.17 110.83,51.14 111.76,52.07 111.76,53.85 112.27,54.36 112.27,60.45 115.6,63.78 X2.L7
M4.ENA
  Top 0.305: MCU1.33 97.54,41.91 98.81,43.18 98.81,50.55 100.7,52.44 IC2.2
M4.ENAO
  Top 0.305: IC2.18 110.74,51.79 111.25,52.3 111.25,54.1 111.76,54.61 111.76,60.71 114.41,63.36 X2.L6
M4.STEP
  Top 0.305: MCU1.31 99.82,42.67 99.82,50.04 100.92,51.14 IC2.4
M4.STEPO
  Top 0.305: IC2.16 110.94,50.49 112.27,51.82 112.27,53.59 112.78,54.1 112.78,58.65 X2.L8
M5.DIR
  Top 0.305: MCU1.38 95.25,50.8 97.54,50.8 100.33,53.59 100.33,60.45 101.15,61.27 IC1.6
M5.DIRO
  Top 0.305: IC1.14 110.15,60.62 111.76,62.23 111.76,80.78 112.27,81.28 X2.L2
M5.ENA
  Top 0.305: MCU1.39 95.25,48.26 93.47,48.26 92.71,49.02 92.71,50.04 93.47,50.8 94.49,50.8 95.25,51.56 95.25,52.58 96.01,53.34 99.31,53.34 99.82,53.85 99.82,60.71 101.04,61.92 IC1.5
M5.ENAO
  Top 0.305: IC1.15 110.04,61.27 111.25,62.48 111.25,84.28 111.76,84.78 X2.L1
M5.STEP
  Top 0.305: MCU1.37 98.3,48.77 98.3,50.8 100.84,53.34 100.84,60.2 101.26,60.62 IC1.7
M5.STEPO
  Top 0.305: IC1.13 110.26,59.97 112.27,61.98 112.27,77.28 112.78,77.78 X2.L3
M6.DIR
  Top 0.305: MCU1.43 95.25,53.34 93.47,53.34 92.71,54.1 92.71,55.12 93.47,55.88 94.49,55.88 95.25,56.64 95.25,57.66 96.01,58.42 98.3,58.42 98.81,58.93 98.81,61.21 100.81,63.22 IC1.3
M6.DIRO
  Top 0.305: IC1.17 109.56,62.57 110.24,63.25 110.24,88.14 109.47,88.9 102.89,88.9 102.38,89.41 X1.L2
M6.ENA
  Top 0.305: MCU1.44 95.25,58.42 95.25,60.45 95.76,60.96 97.79,60.96 100.7,63.87 IC1.2
M6.ENAO
  Top 0.305: IC1.18 109.45,63.22 109.73,63.5 109.73,87.88 109.22,88.39 99.39,88.39 98.88,88.9 X1.L1
M6.STEP
  Top 0.305: MCU1.42 95.25,55.88 98.81,55.88 99.31,56.39 99.31,60.96 100.92,62.57 IC1.4
M6.STEPO
  Top 0.305: IC1.16 109.93,61.92 110.74,62.74 110.74,88.39 109.73,89.41 106.39,89.41 105.88,89.92 X1.L3
N$2
  Top 0.305: R46.1 82.55,14.59 Q16.6 Q16.5
N$3
  Top 0.305: Q16.4 84.26,15.89 84.45,15.7 84.45,15.43 84.64,15.24 Q16.2 85.67,15.24 86.17,15.74 R62.2
N$4
  Top 0.305: Q16.3 85.36,15.89 85.72,16.26 OC21.2
N$5
  Top 0.305: R45.1 76.83,14.59 Q15.6 Q15.5
N$6
  Top 0.305: Q15.4 78.55,15.89 78.74,15.7 78.74,15.43 78.93,15.24 Q15.2 79.96,15.24 80.46,15.74 R61.2
N$7
  Top 0.305: Q15.3 79.64,15.89 80.01,16.26 OC20.2
N$8
  Top 0.305: R44.1 71.12,14.59 Q14.6 Q14.5
N$9
  Top 0.305: Q14.4 72.83,15.89 73.03,15.7 73.03,15.43 73.22,15.24 Q14.2 74.24,15.24 74.74,15.74 R60.2
N$10
  Top 0.305: Q14.3 73.93,15.89 74.3,16.26 OC19.2
N$11
  Top 0.305: R43.1 65.41,14.59 Q13.6 Q13.5
N$12
  Top 0.305: Q13.4 67.12,15.89 67.31,15.7 67.31,15.43 67.5,15.24 Q13.2 68.53,15.24 69.03,15.74 R59.2
N$13
  Top 0.305: Q13.3 68.21,15.89 68.58,16.26 OC18.2
N$14
  Top 0.305: R42.1 59.69,14.59 Q12.6 Q12.5
N$15
  Top 0.305: Q12.4 61.4,15.89 61.59,15.7 61.59,15.43 61.78,15.24 Q12.2 62.81,15.24 63.31,15.74 R58.2
N$16
  Top 0.305: Q12.3 62.5,15.89 62.87,16.26 OC17.2
N$17
  Top 0.305: R41.1 53.98,14.59 Q11.6 Q11.5
N$18
  Top 0.305: Q11.4 55.69,15.89 55.88,15.7 55.88,15.43 56.07,15.24 Q11.2 57.1,15.24 57.6,15.74 R57.2
N$19
  Top 0.305: Q10.3 84.19,85.71 83.82,85.34 OC15.2
N$20
  Top 0.305: R40.1 87,87.01 Q10.6 Q10.5
N$21
  Top 0.305: Q10.4 85.28,85.71 85.09,85.9 85.09,86.17 84.9,86.36 Q10.2 83.87,86.36 83.37,85.86 R56.2
N$22
  Top 0.305: Q11.3 56.78,15.89 57.15,16.26 OC16.2
N$23
  Top 0.305: R34.1 52.7,87.01 Q4.6 Q4.5
N$24
  Top 0.305: R39.1 81.28,87.01 Q9.6 Q9.5
N$25
  Top 0.305: Q9.4 79.57,85.71 79.38,85.9 79.38,86.17 79.18,86.36 Q9.2 78.16,86.36 77.66,85.86 R55.2
N$26
  Top 0.305: R18.2 R21.1 30.86,17.53 30.35,18.04 30.35,22.1 30.86,22.61 34.04,22.61 34.54,23.11 OC4.3
N$27
  Top 0.305: R24.1 R22.2 40.51,18.53 40.01,18.03 40.01,16.97 39.18,16.14 C5.1
N$28
  Top 0.305: Q9.3 78.47,85.71 78.11,85.34 OC14.2
N$29
  Top 0.305: R38.1 75.56,87.01 Q8.6 Q8.5
N$30
  Top 0.305: Q8.4 73.85,85.71 73.66,85.9 73.66,86.17 73.47,86.36 Q8.2 72.44,86.36 71.94,85.86 R54.2
N$31
  Top 0.305: C4.1 32.89,16.76 33.4,17.27 34.61,17.27 34.92,17.59 34.92,18.22 34.61,18.54 31.11,18.54 R21.2 R23.1
N$32
  Top 0.305: C6.1 34.42,16.26 35.43,17.27 35.43,18.54 34.8,19.18 IC5.3 32.64,19.18 31.88,19.94 31.88,20.83 31.63,21.07 R23.2
N$33
  Top 0.305: Q8.3 72.76,85.71 72.39,85.34 OC13.2
N$34
  Top 0.305: R37.1 69.85,87.01 Q7.6 Q7.5
N$35
  Top 0.305: Q7.4 68.14,85.71 67.94,85.9 67.94,86.17 67.75,86.36 Q7.2 66.73,86.36 66.23,85.86 R53.2
N$36
  Top 0.305: C7.1 37.47,17.91 IC5.5 39.18,18.54 39.77,18.54 40.01,18.77 40.01,20.57 40.51,21.07 R24.2
N$37
  Top 0.305: OC4.1 49.65,20.57 R11.2
N$38
  Top 0.305: Q7.3 67.04,85.71 66.67,85.34 OC12.2
N$39
  Top 0.305: R36.1 64.14,87.01 Q6.6 Q6.5
N$40
  Top 0.305: Q6.4 62.42,85.71 62.23,85.9 62.23,86.17 62.04,86.36 Q6.2 61.01,86.36 60.51,85.86 R52.2
N$41
  Top 0.305: R19.2 R22.1 OC5.3
N$42
  Top 0.305: OC5.1 49.65,14.99 R12.2
N$43
  Top 0.305: Q6.3 61.33,85.71 60.96,85.34 OC11.2
N$44
  Top 0.305: R35.1 58.42,87.01 Q5.6 Q5.5
N$45
  Top 0.305: Q5.4 56.71,85.71 56.52,85.9 56.52,86.17 56.33,86.36 Q5.2 55.3,86.36 54.8,85.86 R51.2
N$46
  Top 0.305: Q4.4 50.99,85.71 50.8,85.9 50.8,86.17 50.61,86.36 Q4.2 49.58,86.36 49.08,85.86 R50.2
N$47
  Top 0.305: Q4.3 49.9,85.71 49.53,85.34 OC9.2
N$48
  Top 0.305: Q5.3 55.61,85.71 55.24,85.34 OC10.2
N$49
  Top 0.305: R33.1 46.99,87.01 Q3.6 Q3.5
N$50
  Top 0.305: Q3.4 45.28,85.71 45.09,85.9 45.09,86.17 44.9,86.36 Q3.2 43.87,86.36 43.37,85.86 R49.2
N$51
  Top 0.305: Q3.3 44.18,85.71 43.81,85.34 OC8.2
N$52
  Top 0.305: R32.1 41.27,87.01 Q2.6 Q2.5
N$53
  Top 0.305: Q2.4 39.56,85.71 39.37,85.9 39.37,86.17 39.18,86.36 Q2.2 38.15,86.36 37.65,85.86 R48.2
N$54
  Top 0.305: Q2.3 38.47,85.71 38.1,85.34 OC7.2
N$55
  Top 0.305: Q1.5 Q1.6 35.56,87.01 R31.1
N$56
  Top 0.305: R47.2 31.94,85.86 32.44,86.36 Q1.2 33.47,86.36 33.66,86.17 33.66,85.9 33.85,85.71 Q1.4
N$57
  Top 0.305: OC6.2 32.38,85.34 32.75,85.71 Q1.3
N$58
  Top 0.305: R1.2 13.98,24 14.49,23.5 OC1.1
N$59
  Top 0.305: R2.2 7.11,22.86 7.62,22.35 9.91,22.35 10.67,23.11 OC2.1
N$60
  Top 0.305: R3.2 5.59,24 OC3.1
N$61
  Top 0.305: R4.1 15.75,15.91 OC1.4
N$62
  Top 0.305: R5.1 10.67,15.91 OC2.4
N$63
  Top 0.305: R6.1 5.59,15.91 OC3.4
N$64
  Top 0.305: Q17.1 9.4,24 8.89,23.5 OC2.2
N$65
  Top 0.305: Q17.2 11.18,26.91 R63.2
N$66
  Top 0.457: D1.A 16.98,81.28 X8.1
O1
  Top 0.457: IC4.12 25.65,18.8 26.42,18.03 26.42,14.48 25.15,13.21 20.83,13.21 20.32,12.7 20.32,5.56 19.81,5.05 X4.L3
O2
  Top 0.457: IC4.13 25.65,20.07 27.18,18.54 27.18,13.97 25.65,12.45 22.59,12.45 22.08,11.94 X4.L2
O3
  Top 0.457: IC4.14 25.65,21.34 27.94,19.05 27.94,13.46 25.58,11.1 X4.L1
RESET
  Top 0.305: R10.1 31.75,73.66 MCU1.RESET 33.02,76.45 | C21.1 31.82,76.45 33.02,76.45 | OC6.4 34.92,77.6 33.78,76.45 33.02,76.45
RESET+
  Top 0.305: R31.2 35.56,85.34 34.92,84.71 OC6.1
  Top 0.318: X6.L2 27.3,88.14 27.81,87.63 36.01,87.63 36.51,87.12 36.51,86.24 36.13,85.86 R31.2
RESET-
  Top 0.305: Q1.1 31.75,87.01 R47.1 24.31,86.86 23.8,87.37 X6.L1
S.RESET+
  Top 0.305: R32.2 41.27,85.34 40.64,84.71 OC7.1
  Top 0.318: X6.L4 34.3,89.15 34.81,88.65 41.72,88.65 42.23,88.14 42.23,86.24 41.85,85.86 R32.2
S.RESET-
  Top 0.305: Q2.1 37.47,87.01 R48.1
  Top 0.318: R48.1 37.47,87 36.32,88.14 31.31,88.14 30.8,88.65 X6.L3
SOFT.RESET
  Top 0.305: R9.1 52.07,73.66 MCU1.A0 49.78,75.95 47.24,75.95 46.74,76.45 40.64,76.45 | OC7.4 40.64,76.45 | C22.1 37.54,76.45 40.64,76.45
SPIN.DIR
  Top 0.305: MCU1.13 27.69,27.94 12.95,27.94 12.45,27.43 12.45,26.04 11.82,25.41 R63.1
SPIN.ENABLE
  Top 0.305: MCU1.12 30.23,25.4 15.61,25.4 R1.1
SPIN.PWM
  Top 0.305: R12.1 50.42,19.81 51.18,20.57 51.18,23.62 50.16,24.64 43.94,24.64 43.43,25.15 43.43,27.69 42.67,28.45 35.81,28.45 MCU1.11
SPIN.PWM2
  Top 0.305: R11.1 50.42,23.62 49.91,24.13 43.69,24.13 42.93,24.89 42.93,27.43 42.42,27.94 40.39,27.94 MCU1.9
VIN  (via drill 0.35)
  Top 0.457: D1.C v29.21,81.28
  Bottom 0.457: MCU1.VIN 45.72,80.68 45.12,81.28 v29.21,81.28
X.MAX
  Top 0.305: 64.45,24.89 67.56,24.89 68.07,25.4 69.85,25.4 MCU1.RX3 72.39,27.94 R17.1 | OC17.4 60.33,24 61.21,24.89 64.39,24.89 64.45,24.89 | C10.1 64.45,24.89
X.MAX+
  Top 0.305: OC17.1 60.33,16.89 59.69,16.26 R42.2 59.12,15.74 58.74,15.36 58.74,14.48 59.24,13.97 59.8,13.97 60.3,13.46 X7.L10
X.MAX-
  Top 0.305: Q12.1 63.5,14.59 R58.1 63.8,14.74 X7.L9
X.MIN
  Top 0.305: OC16.4 54.61,23.88 55.63,24.89 58.67,24.89 58.74,24.89 | 58.74,24.89 60.45,24.89 60.96,25.4 67.31,25.4 MCU1.TX3 69.85,27.94 R20.1 | C9.1 58.74,24.89
X.MIN+
  Top 0.305: OC16.1 54.61,16.89 53.98,16.26 R41.2 53.4,15.74 53.02,15.36 53.02,14.29 53.3,14.01 X7.L12
X.MIN-
  Top 0.305: R57.1 57.78,14.59 Q11.1 56.8,14.59 X7.L11
Y.MAX
  Top 0.305: C12.1 75.88,24.89 | OC19.4 71.75,24 72.64,24.89 75.88,24.89 | 75.88,24.89 76.2,25.21 MCU1.RX2 77.47,27.94 R15.1
Y.MAX+
  Top 0.305: OC19.1 71.75,16.89 71.12,16.26 R44.2 70.55,15.74 70.17,15.36 70.17,14.48 70.67,13.97 73.8,13.97 74.31,13.46 X7.L6
Y.MAX-
  Top 0.305: Q14.1 74.93,14.59 R60.1 74.93,13.97 75.44,13.46 77.3,13.46 77.81,12.95 X7.L5
Y.MIN
  Top 0.305: 70.17,24.89 71.88,24.89 MCU1.TX2 74.93,27.94 R16.1 | OC18.4 66.04,23.88 66.55,24.38 67.82,24.38 68.33,24.89 70.1,24.89 70.17,24.89 | C11.1 70.17,24.89
Y.MIN+
  Top 0.305: OC18.1 66.04,16.89 65.41,16.26 R43.2 64.83,15.74 64.45,15.36 64.45,14.48 64.96,13.97 66.8,13.97 67.31,13.46 X7.L8
Y.MIN-
  Top 0.305: Q13.1 69.22,14.59 | X7.L7 70.81,12.95 70.3,13.46 69.72,13.46 69.22,13.97 69.22,14.59 | R59.1 69.22,14.59
Z.MAX
  Top 0.305: 83.06,24.89 MCU1.RX1 82.55,27.94 R13.1 | 83.06,24.89 83.19,24.77 OC21.4 | C14.1 86.54,24.89 83.06,24.89
Z.MAX+
  Top 0.305: OC21.1 83.19,16.89 82.55,16.26 R46.2 81.98,15.74 81.6,15.36 81.6,14.48 82.11,13.97 87.8,13.97 88.31,13.46 X7.L2
Z.MAX-
  Top 0.305: Q16.1 86.36,14.59 R62.1 91.3,14.74 91.81,14.23 X7.L1
Z.MIN
  Top 0.305: R14.1 80.01,27.94 MCU1.TX1 78.74,24.89 | C13.1 80.83,24.89 78.74,24.89 | OC20.4 77.47,24 78.36,24.89 78.74,24.89
Z.MIN+
  Top 0.305: OC20.1 77.47,16.89 76.83,16.26 R45.2 76.26,15.74 75.88,15.36 75.88,14.48 76.39,13.97 79.84,13.97 81.31,12.51 X7.L4
Z.MIN-
  Top 0.305: Q15.1 80.64,14.59 R61.1 80.64,13.97 81.15,13.46 84.3,13.46 84.81,12.95 X7.L3

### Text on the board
_tsilk: INPUT | 7-12VDC | + - | +RST- | +SRS- | +FHD- | +CST- | +AMN- | +AMX- | +BMN- | +BMX- | +CMN- | +CMX- | M6E | M6D | M6S | GND | +5V | M5E | M5D | HARDWARE DESIGN RJW 2020 | M5S | r1.1 | GND | +5V | M4E | M4D | M4S | GND | +5V | M3E | M3D | M3S | GND | +5V | M2E | M2D | M2S | GND | +5V | +24V | DG | SEN | SDR | COO | +10V | AG | AO1 | AO2 | +XMN- | +XMX- | +YMN- | +YMX- | +ZMN- | +ZMX- | +5V | GND | M1S | M1D | M1E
